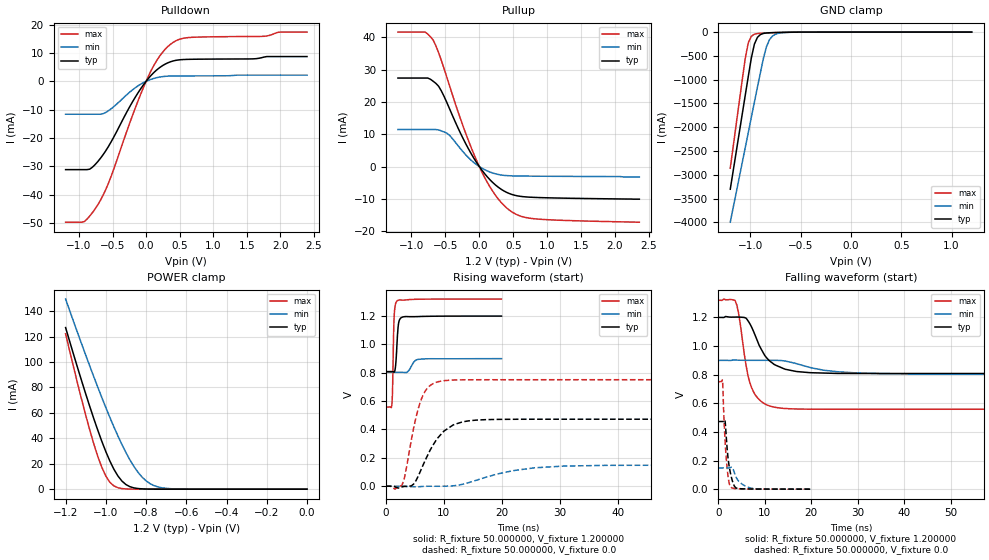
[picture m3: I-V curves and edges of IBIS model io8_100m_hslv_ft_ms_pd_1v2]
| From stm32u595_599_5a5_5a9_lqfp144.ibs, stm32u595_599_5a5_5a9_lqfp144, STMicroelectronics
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|   Model io8_100m_hslv_ft_ms_pd_1v2
[Model]  io8_100m_hslv_ft_ms_pd_1v2
Model_type I/O
Polarity   Non-Inverting
Enable   Active-Low
Vinl =   0.360000V
Vinh =   0.840000V
Vmeas =  0.600000V
Cref =   50.000000pF
Rref =   100.000000M
Vref =   0.0V
C_comp   3.030100pF   2.960800pF   3.078300pF
[Temperature Range]   25.000000   0.140000k   -40.000000
[Pullup Reference]   1.200000V   0.900000V   1.320000V
[Pulldown Reference]   0.0V   0.0V   0.0V
[POWER Clamp Reference]   1.200000V   0.900000V   1.320000V
[GND Clamp Reference]   0.0V   0.0V   0.0V
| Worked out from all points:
|   slope of the pulldown table from 0 to 0.18 V, typ, clamps not added: 40.7 ohm
|   slope of the pullup table from 0 to 0.18 V, typ, clamps not added: 39.5 ohm
|   GND clamp passes 1 mA (typ) near -0.51 V on its own axis
|   POWER clamp passes 1 mA (typ) near -0.86 V on its own axis
|   rising waveform, R_fixture 50.000000, V_fixture 1.200000: 20-80 % time 356ps typ, 873ps min, 231ps max; typ from 0.808 V to 1.2 V
|   rising waveform, R_fixture 50.000000, V_fixture 0.0: 20-80 % time 3.94ns typ, 8.93ns min, 2.36ns max; typ from 0 V to 0.472 V
|   falling waveform, R_fixture 50.000000, V_fixture 1.200000: 20-80 % time 4.09ns typ, 8.68ns min, 2.49ns max; typ from 1.2 V to 0.808 V
|   falling waveform, R_fixture 50.000000, V_fixture 0.0: 20-80 % time 1.04ns typ, 1.96ns min, 796ps max; typ from 0.472 V to 0 V
[Pulldown]
|Voltage   I(typ)   I(min)   I(max)
-1.2V     -31.16mA   -11.61mA   -49.71mA
-920mV    -31.16mA   -11.61mA   -49.48mA
-840mV    -31mA      -11.61mA   -47.54mA
-720mV    -28.33mA   -11.61mA   -43.58mA
-560mV    -22.95mA   -10.37mA   -35.89mA
-200mV    -7.146mA   -2.964mA   -11.89mA
0V        0A         -1pA       0A
160mV     4.047mA    1.298mA    7.361mA
360mV     6.87mA     1.87mA     13mA
640mV     7.765mA    1.923mA    15.46mA
1.76V     8.564mA    2.187mA    15.9mA
2.4V      8.742mA    2.187mA    17.38mA
[Pullup]
|Voltage   I(typ)   I(min)   I(max)
-1.2V     27.42mA    11.47mA    41.66mA
-800mV    27.42mA    11.47mA    41.66mA
-680mV    26.42mA    11.47mA    39.17mA
-600mV    24.87mA    11.36mA    35.26mA
-440mV    17.97mA    9.699mA    25.09mA
-240mV    8.719mA    4.584mA    12.56mA
-40mV     1.247mA    576.2uA    1.879mA
200mV     -4.978mA   -2.01mA    -7.739mA
440mV     -8.335mA   -2.843mA   -13.44mA
600mV     -9.206mA   -2.931mA   -15.29mA
840mV     -9.571mA   -2.98mA    -16.22mA
2.36V     -10.1mA    -3.2mA     -17.23mA
[GND_clamp]
|Voltage   I(typ)   I(min)   I(max)
-1.2V     -3.305A    -3.998A    -2.862A
-1.05V    -1.316A    -2.418A    -539.3mA
-1.02V    -921mA     -2.103A    -218.8mA
-990mV    -539.5mA   -1.788A    -87.45mA
-960mV    -252.2mA   -1.474A    -44.37mA
-930mV    -110.5mA   -1.16A     -30.33mA
-870mV    -28.04mA   -549.1mA   -21.1mA
-840mV    -18.44mA   -305.6mA   -18.29mA
-810mV    -13.92mA   -159.7mA   -15.75mA
-780mV    -11.24mA   -82.36mA   -13.39mA
-600mV    -2.986mA   -4.279mA   -3.072mA
1.2V      30.28uA    18.17uA    37.27uA
[POWER_clamp]
|Voltage   I(typ)   I(min)   I(max)
-1.2V     127mA      149.4mA    122.2mA
-1.12V    84.97mA    114mA      70.27mA
-1.06V    55.51mA    88.42mA    35.67mA
-1.02V    37.63mA    72.04mA    17.17mA
-1V       29.51mA    64.13mA    10.3mA
-960mV    15.69mA    48.99mA    2.571mA
-900mV    3.624mA    28.77mA    182.8uA
-840mV    490.7uA    13.24mA    11.35uA
-800mV    116.8uA    6.532mA    1.77uA
-740mV    13.2uA     1.723mA    109.1nA
-620mV    167.3nA    79.35uA    0A
0V        0A         17.84nA    0A
[Ramp]
| variable   typ   min   max
dV/dt_r  0.28341/3.92317n   88.81788m/8.92178n  0.45046/2.35186n
dV/dt_f  0.23489/4.08024n   58.07400m/8.67612n  0.45673/2.47733n
R_load = 50.000000
[Rising Waveform]
R_fixture= 50.000000
V_fixture= 1.200000
V_fixture_min= 0.900000
V_fixture_max= 1.320000
|time   V(typ)   V(min)   V(max)
0s        808mV      802.7mV    558.2mV
1.041ns   808.4mV    802.7mV    577.4mV
1.161ns   808.1mV    802.7mV    693mV
1.321ns   805.9mV    802.7mV    1.048V
1.441ns   804.2mV    802.7mV    1.203V
1.922ns   1.006V     802.7mV    1.306V
2.242ns   1.159V     802.8mV    1.312V
2.923ns   1.193V     802.6mV    1.312V
5.726ns   1.196V     894.7mV    1.318V
19.94ns   1.199V     899.4mV    1.319V
[Rising Waveform]
R_fixture= 50.000000
V_fixture= 0.0
V_fixture_min= 0.0
V_fixture_max= 0.0
|time   V(typ)   V(min)   V(max)
0s        2.152nV    208.1nV    1.367nV
2.803ns   -4.394mV   53.89uV    8.095mV
3.203ns   -1.38mV    38.77uV    57.99mV
4.805ns   15.36mV    -4.228mV   413.3mV
6.406ns   147.7mV    -1.251mV   642.2mV
8.008ns   281mV      -162.7uV   720.4mV
10.41ns   399.2mV    309.8uV    745.5mV
15.22ns   464.6mV    36.84mV    750.5mV
30.83ns   472.2mV    142mV      750.7mV
199.4ns   472.4mV    148.1mV    750.8mV
[Falling Waveform]
R_fixture= 50.000000
V_fixture= 1.200000
V_fixture_min= 0.900000
V_fixture_max= 1.320000
|time   V(typ)   V(min)   V(max)
0s        1.199V     899.4mV    1.319V
3.604ns   1.202V     901.9mV    1.319V
4.004ns   1.202V     901.2mV    1.286V
6.406ns   1.176V     900mV      790.4mV
7.608ns   1.1V       900mV      678.2mV
10.01ns   933.1mV    900mV      595.4mV
13.21ns   853.7mV    899.1mV    567mV
22.82ns   810.8mV    830.3mV    558.4mV
35.24ns   808mV      806.7mV    558.2mV
199.4ns   808mV      802.7mV    558.2mV
[Falling Waveform]
R_fixture= 50.000000
V_fixture= 0.0
V_fixture_min= 0.0
V_fixture_max= 0.0
|time   V(typ)   V(min)   V(max)
0s        472.4mV    148.1mV    750.8mV
920.9ps   472.7mV    148.2mV    759.7mV
1.201ns   474.2mV    148.2mV    523.8mV
1.441ns   481.6mV    148.2mV    359.5mV
1.682ns   390.7mV    148.2mV    235.8mV
2.242ns   184.3mV    148.1mV    62.43mV
2.723ns   98.56mV    152.7mV    13.9mV
3.764ns   10.32mV    89.86mV    3.558mV
6.767ns   1.547mV    9.869mV    524uV
19.94ns   2.152nV    208.1nV    1.367nV
